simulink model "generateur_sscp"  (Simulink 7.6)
settings: Solver=ode45  StartTime=0.0  StopTime=3  RelTol=1e-3
libraries: nesl_utility x2, MaLibrairieElectrical_lib x1

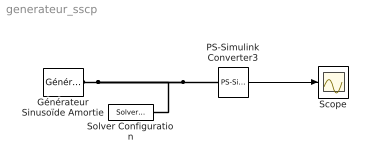
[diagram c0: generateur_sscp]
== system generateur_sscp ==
  Générateur Sinusoïde Amortie : MaLibrairieElectrical_lib/Générateur Sinusoïde Amortie  DialogController=NetworkEngine.DynNeDlgSource  SystemSampleTime=-1  biais=0  w=20 1/s  Amp=1  phi=0 rad  a=2  LocalVarLogging=[]
  PS-Simulink Converter3 : nesl_utility/PS-Simulink Converter  DialogController=NetworkEngine.DynNeUtilDlgSource  SystemSampleTime=-1  PhysicalDomain=network_engine_domain  LeftPortType=input  RightPortType=output  SubClassName=ps_output  Unit=1  AffineConversion=off
  Scope : Scope
  Solver Configuration : nesl_utility/Solver Configuration  DialogController=NetworkEngine.DynNeUtilDlgSource  SystemSampleTime=-1  PhysicalDomain=network_engine_domain  LeftPortType=input  RightPortType=generic  SubClassName=solver  Accelerate=off  Profile=off  ResidualTolerance=1e-9  MaxNonlinIter=3  MaxModeIter=2  DoFixedCost=off  UseLocalSampling=off  DoDC=off  LinearAlgebra=Sparse  LocalSolverSampleTime=.001  LocalSolverChoice=NE_BACKWARD_EULER_ADVANCER  UseLocalSolver=off
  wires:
  PS-Simulink Converter3/1 -> Scope/1
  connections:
  Générateur Sinusoïde Amortie/RConn1 -- PS-Simulink Converter3/LConn1 -- Solver Configuration/RConn1
